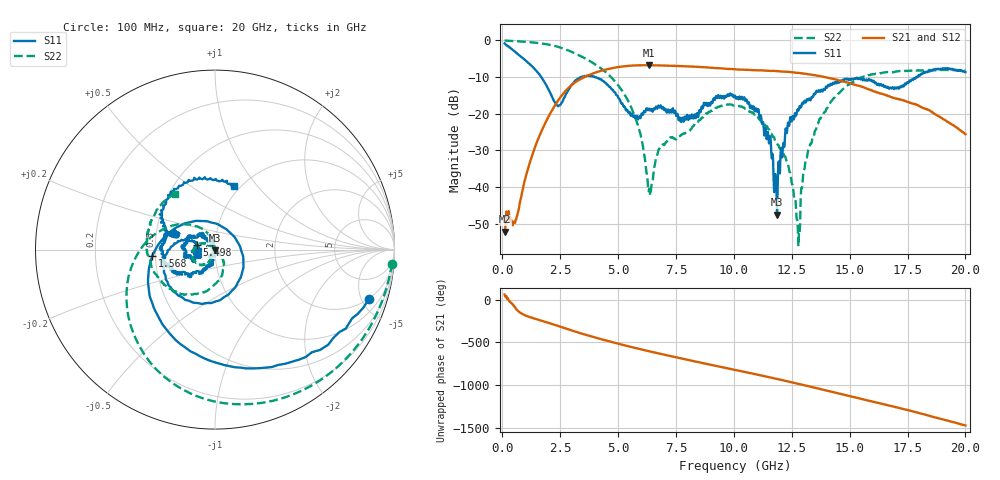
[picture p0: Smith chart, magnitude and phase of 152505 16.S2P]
!  2-Port S-parameters saved by WinCal
! VAR MeasName=S-Parameters (CALIBRATED_DATA) read from VNA (N5230C)
! VAR MeasDate=4/10/2015 9:29:54 AM
! VAR NAME=152505 16
! VAR FILENAME=152505 16.S2P
! VAR DATE=4/10/2015 9:29:54 AM
! VAR PHYS_PORTS=1,2
# Hz S DB R 50
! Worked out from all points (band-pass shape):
!   801 points, 100 MHz to 20 GHz, reference 50 ohm
!   highest |S21| = -6.82 dB at 6.319 GHz (marker M1); lowest = -52.2 dB at 100 MHz (marker M2)
!   |S21| within 3 dB of the highest: 3.621 GHz to 13.75 GHz (10.13 GHz wide, 117 % of centre)
!   lowest |S11| = -47.5 dB at 11.87 GHz (marker M3), VSWR 1.01, Z = 50.1 - j0.416 ohm
!   |S11| at or under -10 dB: 1.677 GHz to 3.431 GHz (1.754 GHz wide, 68.7 % of centre); 3.98 GHz to 17.88 GHz (13.9 GHz wide, 127 % of centre); 17.91333 GHz to 17.9461 GHz (32.77 MHz wide, 0.183 % of centre)
!   |S22| runs from -56.1 to -0.1 dB; largest |S21 - S12| = 0.007
!   S11 on the Smith chart (normalised r, x): 100 MHz: 1.97, -5.79; 1.568 GHz: 0.48, -0.04; 5.498 GHz: 0.81, +0.04; 20 GHz: 0.93, +0.76
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1e8  -0.89 -17.6  -52.21 59.6  -51.94 56.3  -0.08 -4.6
6.22375e8  -3.54 -80.4  -48.15 -115.5  -48.06 -114.2  -0.30 -25.3
1.567625e9  -9.07 -174.0  -26.64 123.6  -26.65 123.7  -0.79 -63.8
2.413375e9  -18.00 46.2  -16.43 52.7  -16.45 52.8  -1.83 -100.4
3.43325e9  -9.99 -110.4  -10.43 -37.3  -10.39 -37.0  -4.49 -144.9
4.403375e9  -11.45 -175.7  -8.10 -111.6  -8.09 -111.7  -8.39 172.7
5.497875e9  -19.57 166.0  -6.97 172.2  -6.96 171.9  -17.38 121.5
5.9705e9  -21.25 -176.7  -6.84 140.7  -6.83 140.8  -25.66 103.8
6.31875e9  -18.68 -167.8  -6.82 118.7  -6.84 118.4  -41.11 141.8
6.741625e9  -17.82 -176.7  -6.88 92.5  -6.87 92.2  -29.99 -127.5
8.283875e9  -20.42 -158.9  -7.22 0.9  -7.23 1.0  -23.17 -115.5
1.005e10  -15.09 169.7  -7.93 -100.7  -7.95 -100.9  -17.87 -166.6
1.106988e10  -18.95 134.2  -8.22 -159.0  -8.19 -159.2  -21.38 156.2
1.186588e10  -47.54 -81.9  -8.42 153.6  -8.46 153.7  -28.18 142.6
1.236338e10  -22.89 -99.3  -8.63 123.0  -8.69 122.9  -34.64 153.7
1.276138e10  -18.83 -112.9  -8.91 98.4  -8.90 98.2  -50.86 165.1
1.308475e10  -16.86 -117.9  -9.16 77.6  -9.18 77.5  -33.28 -37.7
1.338325e10  -15.46 -128.8  -9.44 58.9  -9.39 58.9  -26.99 -47.3
1.475138e10  -10.90 -165.8  -11.30 -29.5  -11.28 -30.3  -13.13 -97.6
1.669162e10  -13.18 157.9  -15.22 -155.5  -15.31 -156.2  -8.72 -165.3
1.83085e10  -8.59 144.0  -18.84 93.6  -18.67 92.1  -8.21 157.0
2e10  -8.72 73.6  -25.63 -29.5  -25.64 -29.1  -8.35 125.9
